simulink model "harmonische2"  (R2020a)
settings: Solver=ode45  StartTime=-8  StopTime=8  MaxStep=0.01  RelTol=1e-3  EnableMultiTasking=on

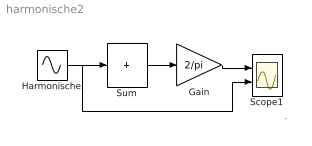
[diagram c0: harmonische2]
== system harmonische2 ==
  note: .
  Gain : Gain  Gain=2/pi  SaturateOnIntegerOverflow=on
  Harmonische : Sin  Amplitude=1./(1:5)  Frequency=1:5  SampleTime=0
  Scope1 : Scope  NumInputPorts=2
  Sum : Sum  Inputs=+  SaturateOnIntegerOverflow=on
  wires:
  Sum/1 -> Gain/1
  Harmonische/1 -> Sum/1, Scope1/2
  Gain/1 -> Scope1/1
